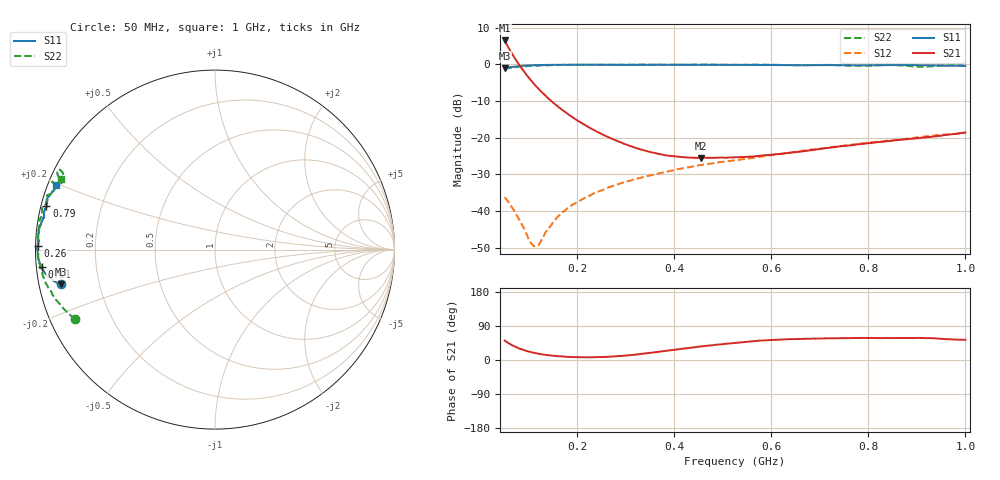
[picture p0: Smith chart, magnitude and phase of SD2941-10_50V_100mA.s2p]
!Agilent Technologies,E8358A,US42080673,A.04.86
!Agilent E8358A: A.04.86
!Date: Friday, June 09, 2006 14:40:12
!Correction: S11(Full 2 Port SOLT,1,2) S21(Full 2 Port SOLT,1,2) S12(Full 2 Port SOLT,1,2) S22(Full 2 Port SOLT,1,2)
!S2P File: Measurements: S11, S21, S12, S22:
# Hz S  MA  R 50
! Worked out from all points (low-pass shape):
!   191 points, 50 MHz to 1 GHz, reference 50 ohm
!   highest |S21| = 6.51 dB at 50 MHz (marker M1); lowest = -25.5 dB at 455 MHz (marker M2)
!   |S21| within 3 dB of the highest: start of sweep to 62.57 MHz
!   lowest |S11| = -1.1 dB at 50 MHz (marker M3), VSWR 15.45, Z = 3.28 - j5.55 ohm
!   |S11| at or under -10 dB: nowhere
!   |S22| runs from -1.2 to -0.1 dB; largest |S21 - S12| = 2.1
!   S11 on the Smith chart (normalised r, x): 50 MHz: 0.07, -0.11; 110 MHz: 0.01, -0.05; 260 MHz: 0.01, +0.01; 790 MHz: 0.02, +0.13; 1 GHz: 0.02, +0.20
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5e7  0.8784 -167.3  2.117 51.3  0.01543 -28.0  0.8716 -153.6
5.5e7  0.8969 -168.0  1.83 47.1  0.01405 -30.4  0.8843 -155.6
6e7  0.9086 -168.6  1.601 43.0  0.01267 -32.8  0.8943 -157.1
6.5e7  0.9203 -169.3  1.408 39.3  0.0112 -34.6  0.9058 -158.6
7.5e7  0.938 -170.6  1.103 33.2  0.008725 -34.2  0.9207 -161.3
9e7  0.9586 -172.3  0.7967 25.9  0.005781 -26.7  0.9402 -164.5
1e8  0.9667 -173.3  0.656 22.2  0.004014 -13.9  0.948 -166.3
1.1e8  0.9714 -174.2  0.5474 19.1  0.003313 12.6  0.9554 -167.9
1.2e8  0.9756 -175.1  0.4632 16.4  0.00343 40.8  0.9628 -169.3
1.35e8  0.9806 -176.1  0.369 13.3  0.005208 64.3  0.9696 -171.2
1.6e8  0.9841 -177.5  0.2653 10.0  0.008415 78.6  0.9786 -174.0
2.1e8  0.9893 -179.4  0.1561 7.3  0.01446 82.0  0.9873 -177.6
2.6e8  0.9881 178.7  0.1042 8.4  0.02042 82.3  0.9887 179.6
3.7e8  0.9879 176.0  0.05961 22.1  0.03289 79.9  0.9888 174.3
4.55e8  0.9854 173.8  0.05287 35.8  0.04219 76.2  0.9919 170.7
5.25e8  0.985 172.4  0.05378 44.9  0.04913 74.1  0.982 168.6
6.85e8  0.9725 168.5  0.06786 56.5  0.0691 70.1  0.9776 162.9
7.9e8  0.9699 165.5  0.08258 58.3  0.08413 66.8  0.9554 159.1
8.45e8  0.9767 164.0  0.0902 57.8  0.09143 65.2  0.9814 157.4
8.9e8  0.9771 162.7  0.09662 58.5  0.09863 63.6  0.9403 157.2
9.6e8  0.9589 159.9  0.1091 55.1  0.1104 61.2  0.9775 152.8
1e9  0.9569 157.8  0.1178 53.4  0.1164 57.6  0.9461 155.3
